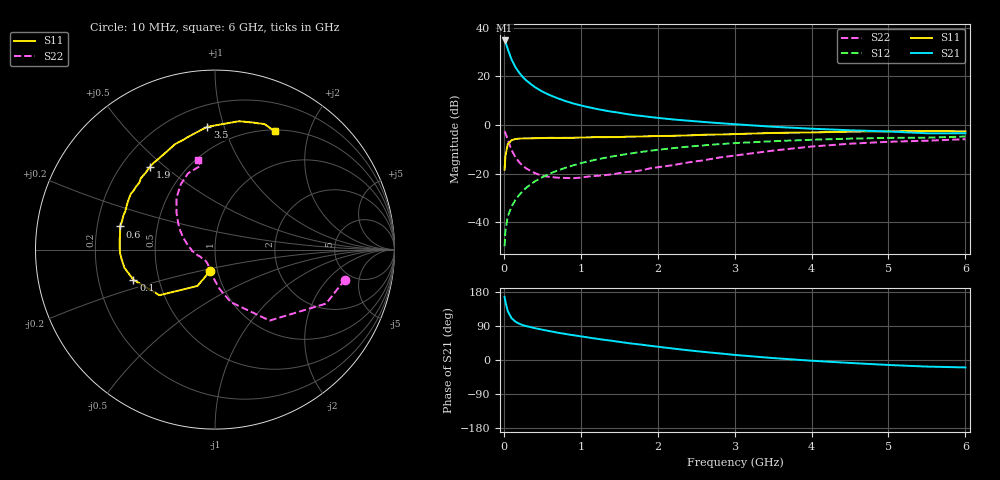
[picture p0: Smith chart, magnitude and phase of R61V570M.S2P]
! SIEMENS Small Signal Semiconductors
! BFR193
! Si NPN RF Bipolar Junction Transistor in SOT23
! VCE = 1.5 V  IC = 70 mA
! Common Emitter S-Parameters:  May  1996
# GHz  S  MA  R  50
!  f  S11  S21  S12  S22
! GHz  MAG  ANG  MAG  ANG  MAG  ANG  MAG  ANG
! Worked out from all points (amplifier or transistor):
!   36 points, 10 MHz to 6 GHz, reference 50 ohm
!   highest |S21| = 34.8 dB at 10 MHz (marker M1)
!   |S21| within 3 dB of that: start of sweep to 45.37 MHz
!   unconditionally stable (mu >= 1): start of sweep to 13.67 MHz; 192.6 MHz to 2.442 GHz
!   at 250 MHz: K = 1.03, MAG = 22.2 dB, |S12| = -27.1 dB
!   at 1.4 GHz: K = 1.05, MAG = 7.9 dB, |S12| = -13.0 dB
!   at 6 GHz: K = 1.00, MSG = 0.7 dB, |S12| = -4.8 dB
!   S11 on the Smith chart (normalised r, x): 10 MHz: 0.92, -0.22; 100 MHz: 0.36, -0.16; 600 MHz: 0.30, +0.11; 1.9 GHz: 0.32, +0.45; 3.5 GHz: 0.34, +0.88; 6 GHz: 0.52, +1.50
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0.01  0.1207 -102.6  54.9 166.5  0.0032 73.3  0.7428 -13.0
0.02  0.225 -115.8  51.28 154.2  0.0065 73.3  0.6882 -25.9
0.05  0.4004 -140.6  36.95 129.2  0.013 66.7  0.4991 -52.4
0.1  0.4846 -159.7  22.25 110.4  0.0209 68.6  0.3055 -73.3
0.15  0.5145 -168.6  15.59 101.2  0.0285 71.2  0.2185 -83.7
0.2  0.5226 -173.8  11.89 95.7  0.0363 72.4  0.1713 -90.4
0.25  0.5292 -177.8  9.546 91.8  0.0444 73.7  0.1417 -96.6
0.3  0.5307 179.3  8.029 89.0  0.0524 74.3  0.1251 -100.4
0.4  0.5338 173.9  6.067 84.2  0.0684 74.7  0.1026 -108.7
0.5  0.537 170.0  4.873 80.0  0.0838 74.1  0.0895 -117.0
0.6  0.5443 166.3  4.097 76.0  0.1 73.2  0.0852 -122.7
0.7  0.5416 163.0  3.542 72.1  0.1159 71.9  0.0822 -127.1
0.8  0.5442 159.9  3.109 68.8  0.1313 70.5  0.0812 -133.1
0.9  0.544 156.3  2.776 65.5  0.1472 69.1  0.0803 -138.7
1.1  0.5561 150.0  2.321 59.3  0.1784 66.1  0.0868 -147.0
1.4  0.5631 141.3  1.878 50.8  0.2234 61.2  0.0961 -158.6
1.9  0.5871 128.1  1.46 37.5  0.2943 52.8  0.1279 -176.6
2.2  0.5978 120.7  1.299 30.2  0.3336 47.6  0.1491 172.8
3.5  0.6853 93.6  0.918 5.1  0.463 25.5  0.2969 136.3
4.5  0.7278 79.4  0.778 -7.8  0.5228 11.2  0.4114 117.5
5.5  0.7519 68.4  0.675 -17.4  0.5475 -2.0  0.4744 99.7
6  0.7382 63.3  0.675 -19.6  0.5779 -6.0  0.5092 100.9
